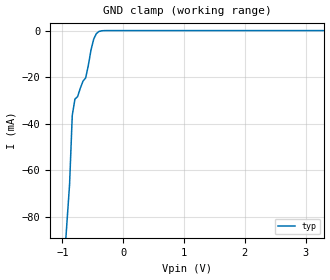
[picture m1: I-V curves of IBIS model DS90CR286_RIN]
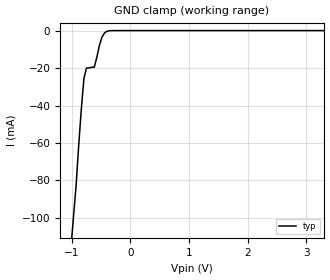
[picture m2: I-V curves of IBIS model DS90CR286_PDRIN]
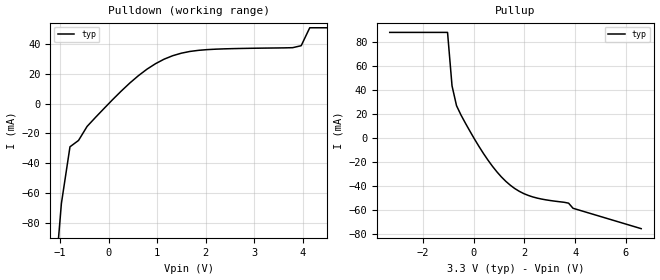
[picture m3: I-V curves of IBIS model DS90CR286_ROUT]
|   National Semiconductor Corporation
|   Interface Products Group
|   IBIS Model of DS90CR286AT-Q1
|   28-Bit LVDS Channel Link Receiver
|   56L TSSOP
[IBIS Ver]   3.2
[Comment char]  |_char
[File name]   ds90cr286at_q1.ibs
[File Rev]   1.2
[Date]   10/07/04
[Source]   File originated at National Semiconductor Corporation.
   Interface Group/Analog Division. All data based on
   Empirical Measurements(Bench).
[Notes]   File created by SBH.
Rev. 1.1:
- updated [Package] and [GND Clamp]-dglisic
Rev. 1.1:
- Changed Vih/Vil for RIN to 100mV
- Changed Vdiff in pin mapping to 200mV
- modified by TSC on 10/31/02
[Disclaimer]
(C) Copyright National Semiconductor Corporation 1994
   All rights reserved
   National Semiconductor Corporation hereby grants
the user of this IBIS model a non-exclusive, nontransferable
license to use this IBIS model under the following terms.
Before using this IBIS model, the user should read this
license.  If the user does not accept these terms,  the
IBIS model should be returned to National within 30 days.
   The user is granted this license only to use the
IBIS model and is not granted rights to sell, load, rent,
lease or license the IBIS model in whole or in part, or in
modified form to anyone other than user. User may modify
the IBIS model to suit its specific applications but rights
to derivative works and such modifications shall belong to
National.
   This IBIS model is provided on an "AS IS" basis and
National makes absolutely no warranty with respect to the
information contained herein.NATIONAL DISCLAIMS AND CUSTOMER
WAIVES ALL WARRANTIES, EXPRESS OR IMPLIED, INCLUDING
WARRANTIES OF MERCHANTABILITY OR FITNESS FOR A PARTICULAR
PURPOSE. The entire risk as to quality and performance is
with the Customer. ACCORDINGLY, IN NO EVENT SHALL THE
COMPANY BE LIABLE FOR ANY DAMAGES, WHETHER IN CONTRACT OR
TORT,INCLUDING ANY LOST PROFITS OR OTHER INCIDENTAL,
CONSEQUENTIAL, EXEMPLARY, OR PUNITIVE DAMAGES ARISING OUT
OF THE USE OR APPLICATION OF THE IBIS model provided in
this package.Further, National reserves the right to make
changes without notice to any product herein to improve
reliability, function, or design. National does not convey
any license under patent rights or any other intellectual
property rights, including those of third parties.
   National is not obligated to provide maintenance or support
for the licensed IBIS model.
Contact National at ATTN:INTERFACE APPLICATIONS/IBIS MODELS.
2900 Semiconductor Drive, M/S A2595, Santa Clara, CA 95052-8090
[Copyright]   Copyright 1994, National Semiconductor, All Rights Reserved
[Component]   DS90CR286MTD
[Manufacturer]  National Semiconductor Corp
[Package]
|   typ   min   max
R_pkg   50.0m   50.0m   50.0m
L_pkg   1.49n   0.95n   2.07n
C_pkg   0.306p   0.146p   0.429p
[Pin]   signal_name   model_name   R_pin   L_pin   C_pin
1   RxOUT22   DS90CR286_ROUT   50.0m   2.07n   0.429p
2   RxOUT23   DS90CR286_ROUT   50.0m   1.49n   0.306p
3   RxOUT24   DS90CR286_ROUT   50.0m   0.95n   0.146p
4   GND   GND   50.0m   0.95n   0.152p
5   RxOUT25   DS90CR286_ROUT   50.0m   0.95n   0.152p
6   RxOUT26   DS90CR286_ROUT   50.0m   0.95n   0.146p
7   RxOUT27   DS90CR286_ROUT   50.0m   1.49n   0.306p
8   LVDSGND   GND   50.0m   2.07n   0.429p
9   RxIN0-   DS90CR286_RIN   50.0m   2.07n   0.429p
10   RxIN0+   DS90CR286_RIN   50.0m   1.49n   0.306p
11   RxIN1-   DS90CR286_RIN   50.0m   0.95n   0.146p
12   RxIN1+   DS90CR286_RIN   50.0m   0.95n   0.152p
13   LVDSVCC   POWER   50.0m   0.95n   0.152p
14   LVDSGND   GND   50.0m   0.95n   0.146p
15   RxIN2-   DS90CR286_RIN   50.0m   1.49n   0.306p
16   RxIN2+   DS90CR286_RIN   50.0m   2.07n   0.429p
17   RxCLKIN-   DS90CR286_RIN   50.0m   2.07n   0.429p
18   RxCLKIN+   DS90CR286_RIN   50.0m   1.49n   0.306p
19   RxIN3-   DS90CR286_RIN   50.0m   0.95n   0.146p
20   RxIN3+   DS90CR286_RIN   50.0m   0.95n   0.152p
21   LVDSGND   GND   50.0m   0.95n   0.152p
22   PLLGND   GND   50.0m   0.95n   0.146p
23   PLLVCC   POWER   50.0m   1.49n   0.306p
24   PLLGND   GND   50.0m   2.07n   0.429p
25   PWRDWN*   DS90CR286_PDRIN   50.0m   2.07n   0.429p
26   RxCLKOUT   DS90CR286_ROUT   50.0m   1.49n   0.306p
27   RxOUT0   DS90CR286_ROUT   50.0m   0.95n   0.146p
28   GND   GND   50.0m   0.95n   0.152p
29   RxOUT1   DS90CR286_ROUT   50.0m   0.95n   0.152p
30   RxOUT2   DS90CR286_ROUT   50.0m   0.95n   0.146p
31   VCC   POWER   50.0m   1.49n   0.306p
32   RxOUT3   DS90CR286_ROUT   50.0m   2.07n   0.429p
33   RxOUT4   DS90CR286_ROUT   50.0m   2.07n   0.429p
34   RxOUT5   DS90CR286_ROUT   50.0m   1.49n   0.306p
35   RxOUT6   DS90CR286_ROUT   50.0m   0.95n   0.146p
36   GND   GND   50.0m   0.95n   0.152p
37   RxOUT7   DS90CR286_ROUT   50.0m   0.95n   0.152p
38   RxOUT8   DS90CR286_ROUT   50.0m   0.95n   0.146p
39   RxOUT9   DS90CR286_ROUT   50.0m   1.49n   0.306p
40   VCC   POWER   50.0m   2.07n   0.429p
41   RxOUT10   DS90CR286_ROUT   50.0m   2.07n   0.429p
42   RxOUT11   DS90CR286_ROUT   50.0m   1.49n   0.306p
43   RxOUT12   DS90CR286_ROUT   50.0m   0.95n   0.146p
44   GND   GND   50.0m   0.95n   0.152p
45   RxOUT13   DS90CR286_ROUT   50.0m   0.95n   0.152p
46   RxOUT14   DS90CR286_ROUT   50.0m   0.95n   0.146p
47   RxOUT15   DS90CR286_ROUT   50.0m   1.49n   0.306p
48   VCC   POWER   50.0m   2.07n   0.429p
49   RxOUT16   DS90CR286_ROUT   50.0m   2.07n   0.429p
50   RxOUT17   DS90CR286_ROUT   50.0m   2.07n   0.429p
51   RxOUT18   DS90CR286_ROUT   50.0m   1.49n   0.306p
52   GND   GND   50.0m   0.95n   0.146p
53   RxOUT19   DS90CR286_ROUT   50.0m   0.95n   0.152p
54   RxOUT20   DS90CR286_ROUT   50.0m   0.95n   0.152p
55   RxOUT21   DS90CR286_ROUT   50.0m   0.95n   0.146p
56   VCC   POWER   50.0m   1.49n   0.306p
[Diff_pin]   inv_pin   vdiff   tdelay_typ   tdelay_min   tdelay_max
| The '+' pin is Diff_pin and the '-' pin is the inv_pin
10   9   .2   0 0 0
12   11   .2   0 0 0
16   15   .2   0 0 0
18   17   .2   0 0 0
20   19   .2   0 0 0
| Models and submodels in the file (3): DS90CR286_RIN (Input), DS90CR286_PDRIN (Input), DS90CR286_ROUT (3-state)
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|   RECEIVER INPUT  MODEL
[Model]   DS90CR286_RIN
Model_type   Input
|Signals   RxIN+,RxIN- ; RxCLKIN+, RxCLKIN-
Vinh = .1
Vinl = -.1
|   typ   min   max
C_comp   5.433pF   NA   NA
|   typ   min   max
[Temperature Range]   25.0   NA   NA
[Voltage range]   3.3V   3.0V   3.6V
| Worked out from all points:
|   GND clamp passes 1 mA (typ) near -0.43 V on its own axis
[Power_clamp]
| Note that the[POWER_clamp]voltage table is referenced to Vcc
| and is calculated using Vtable=Vcc - Vmeasured.
|Voltage   I(typ)   I(min)   I(max)
-3V       0A         NA         NA
0V        0A         NA         NA
[GND_clamp]
|Voltage   I(typ)   I(min)   I(max)
-3.3V     -980mA     NA         NA
-882.3mV  -66.02mA   NA         NA
-838.2mV  -36.43mA   NA         NA
-794.1mV  -29.42mA   NA         NA
-750mV    -28.33mA   NA         NA
-661.8mV  -21.72mA   NA         NA
-617.7mV  -20.31mA   NA         NA
-529.4mV  -8.257mA   NA         NA
-485.3mV  -3.653mA   NA         NA
-441.2mV  -1.289mA   NA         NA
-397.1mV  -352.9uA   NA         NA
3.3V      0A         NA         NA
|   RECEIVER PWRDWN* INPUT MODEL
[Model]   DS90CR286_PDRIN
Model_type   Input
|Signals   PWRDWN*
Vinh = 2.0
Vinl = 0.8
|   typ   min   max
C_comp   5.433pF   NA   NA
|   typ   min   max
[Temperature Range]   25.0   NA   NA
[Voltage range]   3.3V   3.0V   3.6V
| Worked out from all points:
|   GND clamp passes 1 mA (typ) near -0.43 V on its own axis
[GND_clamp]
|Voltage   I(typ)   I(min)   I(max)
-3.3V     -980mA     NA         NA
-926.5mV  -82.06mA   NA         NA
-882.3mV  -60.87mA   NA         NA
-838.2mV  -41.78mA   NA         NA
-794.1mV  -25.51mA   NA         NA
-750mV    -19.98mA   NA         NA
-617.7mV  -19.54mA   NA         NA
-529.4mV  -7.841mA   NA         NA
-485.3mV  -3.454mA   NA         NA
-441.2mV  -1.208mA   NA         NA
-397.1mV  -330.7uA   NA         NA
3.3V      0A         NA         NA
[Power_clamp]
| Note that the[POWER_clamp]voltage table is referenced to Vcc
| and is calculated using Vtable=Vcc - Vmeasured.
|Voltage   I(typ)   I(min)   I(max)
-3.3V     0A         0A         0A
0V        0A         0A         0A
|   RECEIVER OUTPUT  MODEL
[Model]   DS90CR286_ROUT
Model_type   3-state
| Signals   RxOUT0 ~ RxOUT20
Vmeas = 0.0V   |This is 0.0v differential on ouput
Cref = 8pF   |Timing specification test load capacitance value
Vref = 0   |Timing specification test load voltage; GND
| variable   typ   min   max
C_comp   5.247pF   NA   NA
|   typ   min   max
[Temperature Range]   25.0   NA   NA
[Voltage range]   3.3V   3.0V   3.6V
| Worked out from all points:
|   slope of the pulldown table from 0 to 0.495 V, typ, clamps not added: 31.7 ohm
|   slope of the pullup table from 0 to 0.495 V, typ, clamps not added: 29.8 ohm
[Pulldown]
| Voltage   I(typ)   I(min)   I(max)
-3.3V     -980mA     NA         NA
-970.6mV  -67.08mA   NA         NA
-794.1mV  -28.99mA   NA         NA
-617.7mV  -24.71mA   NA         NA
-441.2mV  -15.27mA   NA         NA
441.2mV   14mA       NA         NA
1.147V    30.01mA    NA         NA
1.853V    35.93mA    NA         NA
3.794V    37.72mA    NA         NA
3.971V    39.05mA    NA         NA
4.147V    51.13mA    NA         NA
6.6V      51.13mA    NA         NA
[Pullup]
| Note that the[Pullup]voltage table is referenced to Vcc
| and is calculated using Vtable=Vcc - Vmeasured.
|Voltage   I(typ)   I(min)   I(max)
-3.3V     87.68mA    NA         NA
-1.024V   87.68mA    NA         NA
-847.1mV  43.17mA    NA         NA
-670.6mV  26.7mA     NA         NA
-317.6mV  12.01mA    NA         NA
388.2mV   -13.06mA   NA         NA
917.6mV   -28.37mA   NA         NA
1.447V    -39.55mA   NA         NA
2.329V    -49.29mA   NA         NA
3.741V    -54.49mA   NA         NA
3.918V    -58.76mA   NA         NA
6.6V      -75.72mA   NA         NA
[GND_clamp]
| Outputs in Tri-state.
| Voltage   I(typ)   I(min)   I(max)
| Receiver output is non-tristable
-3V       0A         NA         NA
3V        0A         NA         NA
[POWER_clamp]
| Note that the[POWER_clamp]voltage table is referenced to Vcc
| and is calculated using Vtable=Vcc - Vmeasured.
| Outputs in Tri-state.
|Voltage   I(typ)   I(min)   I(max)
| Receiver output is non-tristable
-3V       0A         NA         NA
0V        0A         NA         NA
[Ramp]
| Note: Ramp rate measured on single-ended Driver Output.
|   typ   min   max
dV/dt_r   3.3/2.625n   NA   NA
dV/dt_f   3.3/2.654n   NA   NA
R_load = 1MOhm  | Represent Hi-Z
